FUNCTION_BLOCK Example10_waituntiltime //4x3 flyways 1 xbots - get xbot status, wait until delay
VAR_INPUT
	Execute : BOOL;
END_VAR
VAR_OUTPUT
	Done : BOOL;
END_VAR
VAR_IN_OUT
	PM_Controller : PMControllerType;	// the planar motor controller to use
END_VAR
VAR
	posX : REAL;
	posY : REAL;
	posZ : REAL;
	posRx : REAL;
	posRy : REAL;
	posRz : REAL;
	xbot_state : USINT;
	cmdlb : UINT;
	PMC_GetXbotStatus1 : PMC_GetXbotStatus;
	PMC_MotionBufferCtrl1 : PMC_MotionBufferCtrl;
	PMC_XYMotion1 : PMC_XYMotion;
	PMC_WaitUntilTimeDelay1 : PMC_WaitUntilTimeDelay; 
	PMC_XYMotion2 : PMC_XYMotion;
	PMC_WaitUntilTimeDelay2 : PMC_WaitUntilTimeDelay;
	PMC_MotionBufferCtrl2 : PMC_MotionBufferCtrl;
END_VAR

//4x3 flyways 1 xbots - get xbot status, wait until delay

//get xbot 1 status
PMC_GetXbotStatus1(Execute := Execute,XbotID := 1,FeedbackType := 0,State => xbot_state,CmdLb => cmdlb,PosX => posX,PosY => posY,PosZ => posZ,PosRx => posRx,PosRy => posRy,PosRz => posRz,PM_Controller := PM_Controller);

//block xbot 1 buffer
PMC_MotionBufferCtrl1(Execute := PMC_GetXbotStatus1.Valid,Level := 0,XbotID := 1,PM_Controller := PM_Controller);

//load move to 900,60
PMC_XYMotion1(Execute := PMC_MotionBufferCtrl1.Done,cmdLB := 3,XbotID := 1,Mode := 0,Type_ := 0,PosX := 0.9,PosY := 0.06,EndVel := 0,MaxVel := 1,MaxAcc := 10,PM_Controller := PM_Controller);

//load wait for 5 seconds
PMC_WaitUntilTimeDelay1(Execute := PMC_XYMotion1.Ack,cmdLB := 4,XbotID := 1,Delay := 5.0,PM_Controller := PM_Controller);

//load move to 60,60
PMC_XYMotion2(Execute := PMC_WaitUntilTimeDelay1.Ack,cmdLB := 5,XbotID := 1,Mode := 0,Type_ := 0,PosX := 0.06,PosY := 0.06,EndVel := 0,MaxVel := 1,MaxAcc := 10,PM_Controller := PM_Controller);

//load wait for 5 seconds
PMC_WaitUntilTimeDelay2(Execute := PMC_XYMotion2.Ack,cmdLB := 6,XbotID := 1,Delay := 5.0,PM_Controller := PM_Controller);

//release xbot 1 buffer
PMC_MotionBufferCtrl2(Execute := PMC_WaitUntilTimeDelay2.Ack,Level := 1,XbotID := 1,PM_Controller := PM_Controller);

Done := PMC_WaitUntilTimeDelay2.Done;

END_FUNCTION_BLOCK
